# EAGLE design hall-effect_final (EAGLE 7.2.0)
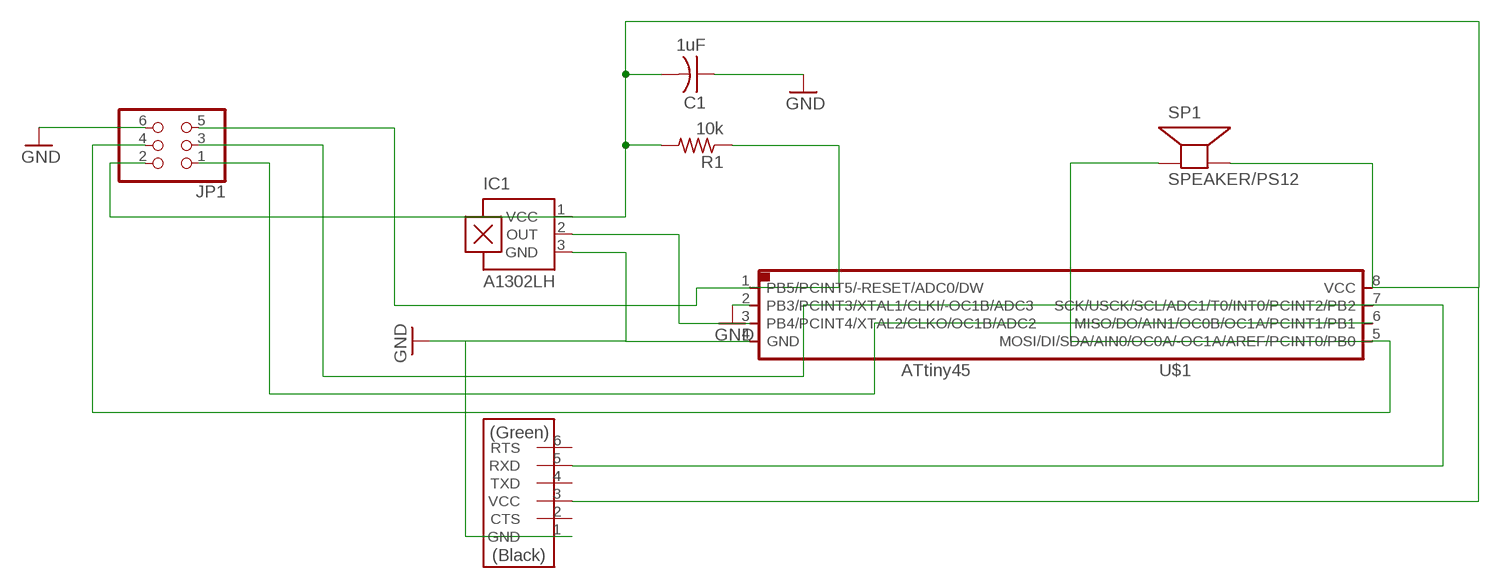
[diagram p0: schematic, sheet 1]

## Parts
C1  1uF  CAP-US1206FAB  [C1206FAB]
IC1  A1302LH  [SOT23-W]
JP1  PINHD-2X3-SMD  [2X03SMD]
R1  10k  RES-US1206FAB  [R1206FAB]
SP1  SPEAKER/PS12  [PS12]
U$1  ATTINY45SI  [SOIC8]
U$2  FTDI-SMD-HEADER  [1X06SMD]

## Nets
GND: C1.1 IC1.3(GND) JP1.6 U$1.2(PB3/PCINT3/XTAL1/CLKI/-OC1B/ADC3) U$1.4(GND) U$2.1(GND)
N$1: C1.2 IC1.1(VCC) JP1.2 R1.2 SP1.P$2(-) U$1.8(VCC) U$2.3(VCC)
N$2: JP1.5 R1.1 U$1.1(PB5/PCINT5/-RESET/ADC0/DW)
N$4: IC1.2(OUT) U$1.3(PB4/PCINT4/XTAL2/CLKO/OC1B/ADC2)
N$5: JP1.3 U$1.7(SCK/USCK/SCL/ADC1/T0/INT0/PCINT2/PB2) U$2.5(RXD)
N$6: JP1.4 SP1.P$1(+) U$1.5(MOSI/DI/SDA/AIN0/OC0A/-OC1A/AREF/PCINT0/PB0)
N$7: JP1.1 U$1.6(MISO/DO/AIN1/OC0B/OC1A/PCINT1/PB1)
Unconnected: U$2.2(CTS) U$2.4(TXD) U$2.6(RTS)

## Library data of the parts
C1 = fab:CAP-US
IC1 = allegro:A13*?: Linear Hall Effect Sensor ICs Continuous-Time Ratiometric High-Temperature Operation Programmable Linear with Analog Output A1302 -Replacement- UGN3503 Source: http://www.allegromicro.com/en/Products/Part_Numbers/1301/1301.pdf http://www.allegromicro.com/en/Products/Part_Numbers/1321/1321.pdf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; MF: ALLEGRO MICROSYSTEMS, INC.; MPN: A1302ELHLT-T; OC_FARNELL: 1457209; OC_NEWARK: 31K6638
JP1 = fab:PINHD-2X3-SMD: PIN HEADER
R1 = fab:RES-US: Resistor (US Symbol)
SP1 = adafruit:SPEAKER: SPEAKER
U$1 = fab:ATTINY45
U$2 = fab:FTDI-SMD-HEADER

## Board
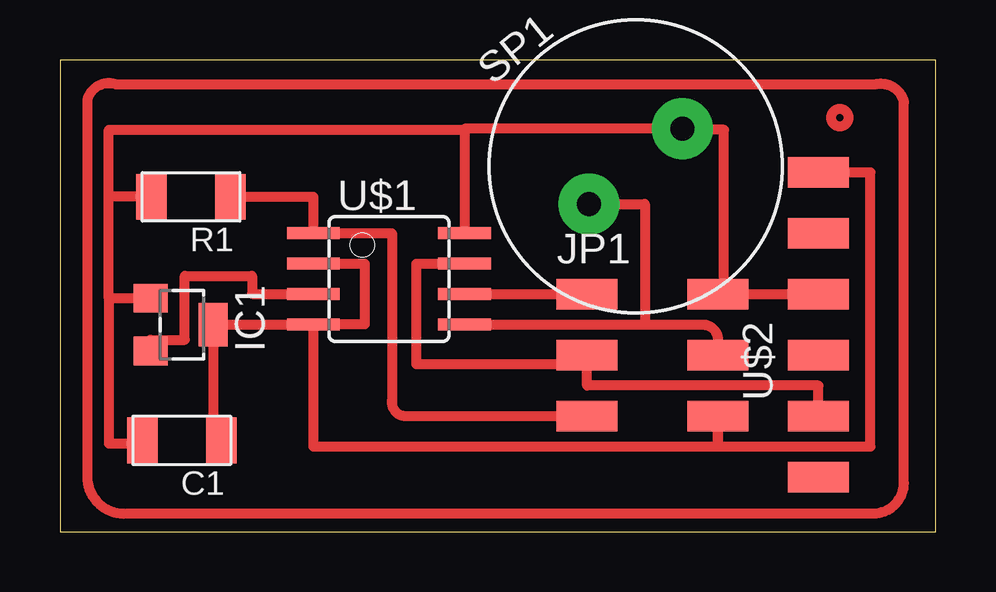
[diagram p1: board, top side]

Size 36.5 x 19.68 mm. Coordinates in mm from the lower left corner, seen from the top.
Outline: 0,0 36.5,0 36.5,19.68 0,19.68 0,0
Copper layers (1*16): Top 0.035mm / dielectric 1.5mm / Bottom 0.035mm
Design rules "default": minimum track width 10mil, minimum drill 24mil, track to track 8mil, track to pad 8mil, pad to pad 8mil, via to via 8mil, smd to smd 8mil, copper to edge 40mil, drill to drill 8mil, minimum pad ring 10mil, minimum via ring 8mil, stop-mask expansion 4mil, vias tented up to drill 0mil, thermal gap 10mil

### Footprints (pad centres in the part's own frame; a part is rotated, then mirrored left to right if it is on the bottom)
C1206FAB = smd 1.27 x 1.905: 1 -1.651,0; 2 1.651,0
SOT23-W = smd 1.2 x 1.4: 1 -1.1,-1.3; 2 1.1,-1.3 | smd 1.8 x 1.2: 3 0,1.3
2X03SMD = smd 2.54 x 1.27: 1 -2.54,2.54; 2 2.92,2.54; 3 -2.54,0; 4 2.92,0; 5 -2.54,-2.54; 6 2.92,-2.54
R1206FAB = smd 1.27 x 1.905: 1 -1.651,0; 2 1.651,0
PS12 = drill 1 pad 2.54: P$1 -2.5,0; P$2 2.5,0
SOIC8 = smd 0.5 x 2.2: 1 -1.905,-3.154; 2 -0.645,-3.154; 3 0.625,-3.154; 4 1.895,-3.154; 5 1.905,3.154; 6 0.635,3.154; 7 -0.635,3.154; 8 -1.905,3.154
1X06SMD = smd 2.54 x 1.27: 1 0,6.35; 2 0,3.81; 3 0,1.27; 4 0,-1.27; 5 0,-3.81; 6 0,-6.35

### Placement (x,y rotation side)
C1  5.08,3.81 180 top
IC1  5.08,8.64 270 top
JP1  24.51,7.37 0 top
R1  5.46,13.97 180 top
SP1  24,15.24 38.9 top
U$1  13.72,10.54 270 top
U$2  31.62,8.64 0 top

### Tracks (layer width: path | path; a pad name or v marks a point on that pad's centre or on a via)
GND
  Top 0.406: U$1.4 IC1.3 6.38,3.05 6.48,3.05 6.48,3.81 C1.1 | U$1.4 10.56,3.56 27.43,3.56 | 27.43,3.56 JP1.6 27.43,3.56 | 27.43,3.56 | 27.43,3.56 33.78,3.56 33.78,14.99 U$2.1 | U$1.2 10.56,11.18 12.7,11.18 12.7,8.65 U$1.4
N$1
  Top 0.406: U$2.3 arc90 32,9.53 32.13,9.53 arc90 31.88,9.91 JP1.2 27.69,9.91 27.69,16.76 25.95,16.76 SP1.P$2 16.87,16.81 16.87,16.76 | 2.03,9.74 2.03,3.68 3.43,3.68 C1.2 | IC1.1 2.03,9.74 | 2.03,9.74 2.03,13.97 | R1.2 2.03,13.97 | 2.03,13.97 2.03,16.76 16.87,16.76 | 16.87,16.76 U$1.8
N$2
  Top 0.406: JP1.5 14.35,4.83 arc-90 13.84,5.46 13.84,12.45 U$1.1 10.56,13.97 R1.1
N$4
  Top 0.406: IC1.2 3.78,8 5.21,8 5.21,10.67 8,10.67 8,9.92 U$1.3
N$5
  Top 0.406: U$2.5 31.62,6.1 21.97,6.1 JP1.3 21.97,6.99 14.86,6.99 14.86,11.18 U$1.7
N$6
  Top 0.406: U$1.5 24.38,8.64 | 24.38,8.64 26.8,8.64 arc-90 27.43,8 JP1.4 | SP1.P$1 24.38,13.67 24.38,8.64
N$7
  Top 0.406: U$1.6 arc90 17,9.91 JP1.1
N$13
  Top 0.406: 2.29,18.67 arc90 1.14,18.03 1.14,2.16 arc90 2.79,0.76 33.91,0.76 arc90 35.18,2.03 35.18,17.91 arc90 34.04,18.67 2.29,18.67
(copper drawn outside any net)
  shapes: Top circle x1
